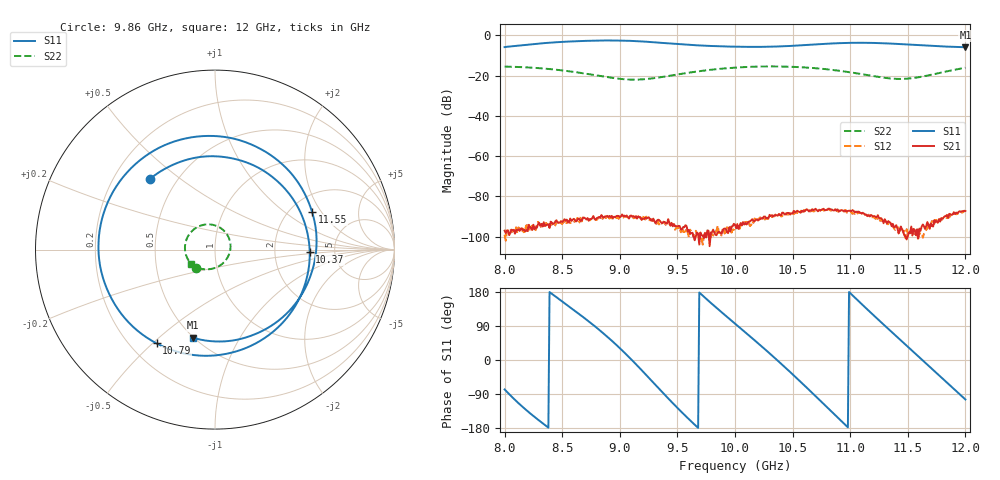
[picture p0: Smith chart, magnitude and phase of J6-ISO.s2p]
!Keysight Technologies,N5234A,MY52241180,A.10.60.03
!Date: Tuesday, May 30, 2023 15:23:29
!Correction: S11(Full 2 Port(1,2))
!S21(Full 2 Port(1,2))
!S12(Full 2 Port(1,2))
!S22(Full 2 Port(1,2))
!S2P File: Measurements: S11, S21, S12, S22:
# Hz S  dB  R 50
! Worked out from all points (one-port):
!   401 points, 8 GHz to 12 GHz, reference 50 ohm
!   lowest |S11| = -5.9 dB at 12 GHz (marker M1), VSWR 3.05, Z = 24.7 - j32.6 ohm
!   |S11| at or under -10 dB: nowhere
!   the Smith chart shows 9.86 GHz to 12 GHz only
!   S11 on the Smith chart (normalised r, x): 9.86 GHz: 0.36, +0.39; 10.37 GHz: 3.23, -0.12; 10.79 GHz: 0.31, -0.51; 11.55 GHz: 2.60, +1.65; 12 GHz: 0.49, -0.65
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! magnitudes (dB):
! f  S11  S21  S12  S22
! 8 GHz  -5.9  -97.0  -99.0  -15.6
! 8.15 GHz  -4.9  -95.8  -97.9  -15.8
! 8.34 GHz  -3.9  -92.8  -94.7  -16.5
! 8.5 GHz  -3.3  -92.6  -93.7  -17.4
! 8.67 GHz  -2.8  -91.7  -92.4  -18.7
! 8.94 GHz  -2.6  -90.7  -90.9  -21.2
! 9.06 GHz  -2.7  -89.5  -90.3  -21.9
! 9.19 GHz  -3.0  -91.7  -91.1  -21.9
! 9.34 GHz  -3.6  -91.6  -93.9  -20.9
! 9.64 GHz  -4.9  -99.8  -100.1  -18.2
! 9.86 GHz  -5.4  -97.6  -98.2  -16.7
! 10 GHz  -5.6  -94.0  -94.5  -16.0
! 10.18 GHz  -5.8  -91.8  -91.5  -15.6
! 10.37 GHz  -5.5  -89.6  -89.6  -15.5
! 10.67 GHz  -4.6  -86.3  -87.1  -16.2
! 10.79 GHz  -4.2  -86.8  -86.8  -16.8
! 11.06 GHz  -3.7  -87.8  -88.8  -18.9
! 11.34 GHz  -4.1  -92.8  -92.6  -21.4
! 11.44 GHz  -4.4  -95.0  -95.6  -21.7
! 11.55 GHz  -4.7  -96.1  -98.5  -21.2
! 11.66 GHz  -5.1  -94.6  -96.6  -20.1
! 12 GHz  -5.9  -87.3  -87.2  -16.1
